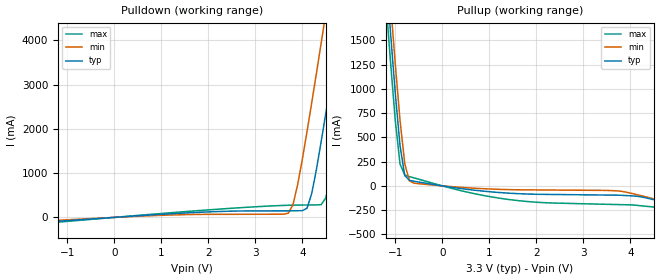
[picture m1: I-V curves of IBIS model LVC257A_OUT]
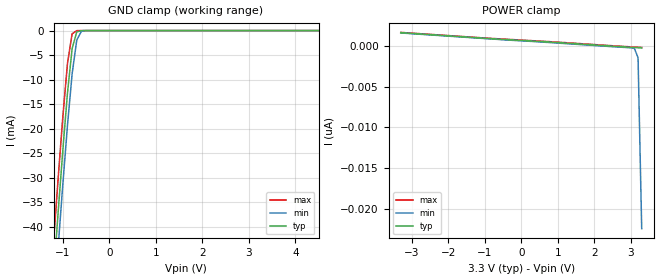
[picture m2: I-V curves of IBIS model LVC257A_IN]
|   TEXAS INSTRUMENTS INCORPORATED
|   Advanced Bus Interface Group
|   IBIS Model of LVC257A
|   Quadruple_2-Line_to_1-Line_Data_Selector/Multiplexer
|   SSOP 16-pin (DB) Package
[IBIS Ver]   2.1
[File Name]   257a.ibs
[File Rev]   1.0
[Date]   11/26/97
[Source]   File originated at Texas Instruments, Inc.
[Notes]   The following is an IBIS list for the LVC257A.
|   - All test data contained in this file are derived from
|   hspice(tm) simulations.
|   - File created by Ramzi Ammar, SLL Applications.
[Disclaimer] Property of Texas Instruments Incorporated.  Unauthorized
   reproduction and/or distribution is strictly prohibited.
   This product is protected under copyright law.
   Created 1997, (C) Copyright 1997, Texas Instruments Inc.,
   All Rights Reserved
   UNLESS THERE IS A SIGNED, WRITTEN AGREEMENT TO THE
   CONTRARY, TEXAS INSTRUMENTS ("TI") IS PROVIDING THE IBIS
   MODELS "AS IS" AND WITHOUT ANY WARRANTY, EXPRESSED OR
   IMPLIED.  TI assumes no liability for:
   1) the accuracy of the IBIS models provided to your
   company;
   2) the proper functioning of these IBIS models in your
   design or for any resulting applications; or
   3) infringement of patents, copyrights or intellectual
   property rights resulting from your use of these IBIS
   models.
   TI provides IBIS Models as a service to our customers.
   You and your company shall not distribute, sell or give
   these models to anyone else without prior written
   permission from TI.
   TI reserves the right to make changes to our products or
   to discontinue any semiconductor product or service
   without notice, and advises our customers to obtain the
   latest version of relevant information to verify, before
   placing orders, that the information being relied on is
   current.
   Please be aware that your receipt and use of the IBIS
   information provided shall serve as acceptance of these
   terms and conditions.  If you do not accept these terms,
   you should return or destroy the IBIS models and any
   other accompanying information immediately.
[Component]   LVC257A
|   (Quadruple_2-Line_to_1-Line_Data_Selector/Multiplexer)
[Manufacturer]  Texas Instruments, Inc.
[Package]
|   typ   min   max
R_pkg   0.033   0.028   0.035
L_pkg   3.97nH   3.65nH   4.58nH
C_pkg   0.34pF   0.31pF   0.37pF
[Pin]   signal_name   model_name   R_pin   L_pin   C_pin
1   A_NOT/B   LVC257A_IN   0.028   4.579nH   0.367pF
2   1A   LVC257A_IN   0.035   4.195nH   0.373pF
3   1B   LVC257A_IN   0.035   3.705nH   0.324pF
4   1Y   LVC257A_OUT   0.032   3.648nH   0.310pF
5   2A   LVC257A_IN   0.032   3.648nH   0.310pF
6   2B   LVC257A_IN   0.035   3.705nH   0.324pF
7   2Y   LVC257A_OUT   0.035   4.195nH   0.373pF
8   GND   GND   0.028   4.579nH   0.367pF
9   3Y   LVC257A_OUT   0.028   4.579nH   0.367pF
10   3B   LVC257A_IN   0.035   4.195nH   0.373pF
11   3A   LVC257A_IN   0.035   3.705nH   0.324pF
12   4Y   LVC257A_OUT   0.032   3.648nH   0.310pF
13   4B   LVC257A_IN   0.032   3.648nH   0.310pF
14   4A   LVC257A_IN   0.035   3.705nH   0.324pF
15   OE_NOT   LVC257A_IN   0.035   4.195nH   0.373pF
16   VCC   POWER   0.028   4.579nH   0.367pF
| Models and submodels in the file (2): LVC257A_OUT (Output), LVC257A_IN (Input)
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|   Model LVC257A_OUT
[Model]   LVC257A_OUT
Model_type   Output
Polarity   Inverting
|variable   typ   min   max
C_comp   5pF   NA   NA
[Voltage range]   3.3   3.0   3.6
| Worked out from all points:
|   slope of the pulldown table from 0 to 0.495 V, typ, clamps not added: 14 ohm
|   slope of the pullup table from 0 to 0.495 V, typ, clamps not added: 14.6 ohm
[Pullup]   | Note: Vtable = Vcc - Voutput
|   Voltage   I(typ)   I(min)   I(max)
-3.3V     16.91A     17.19A     16.64A
-1.2V     2.207A     2.519A     1.903A
-1.1V     1.559A     1.869A     1.259A
-1V       945.7mA    1.245A     664.8mA
-900mV    412.4mA    673.4mA    224.1mA
-800mV    106.4mA    228.5mA    111.8mA
-700mV    56.81mA    49.85mA    95.57mA
-600mV    47.48mA    27.69mA    82.06mA
1.4V      -74.65mA   -38.4mA    -139.4mA
3.8V      -96.78mA   -55.41mA   -193.4mA
4.7V      -166.8mA   -158.7mA   -231.5mA
6.6V      -409.3mA   -400.4mA   -477.6mA
[Pulldown]
|   Voltage   I(typ)   I(min)   I(max)
-3.3V     -302.9mA   -307.1mA   -301.8mA
-1.2V     -88.83mA   -65.71mA   -108.2mA
3.7V      148.2mA    92.73mA    273.4mA
3.8V      148.6mA    281.9mA    276.3mA
3.9V      149mA      735.6mA    278.3mA
4.1V      206.1mA    1.937A     279.8mA
4.2V      538.9mA    2.588A     280.4mA
4.4V      1.702A     3.929A     287.2mA
4.5V      2.352A     4.611A     438.2mA
4.8V      4.382A     6.685A     2.176A
5.1V      6.463A     8.781A     4.214A
6.6V      17.07A     19.4A      14.8A
[Ramp]
| variable   typ   min   max
dV/dt_r   1.5182E+00/3.1012E-10  1.0921E+00/4.4177E-10  1.8637E+00/2.2885E-10
dV/dt_f   1.5740E+00/2.6661E-10  1.3168E+00/3.2470E-10  1.7802E+00/2.0785E-10
|   Model LVC257A_IN
[Model]   LVC257A_IN
Model_type   Input
Polarity   Inverting
Vinl = 0.8V
Vinh = 2.0V
|variable   typ   min   max
C_comp   5pF   NA   NA
[Voltage Range]   3.3   3.0   3.6
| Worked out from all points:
|   GND clamp passes 1 mA (typ) near -0.72 V on its own axis
[POWER_Clamp]   | Note: Vtable = Vcc - Voutput
|   Voltage   I(typ)   I(min)   I(max)
-3.3V     1.569nA    1.537nA    1.605nA
3.1V      -240.8pA   -356.4pA   -183.8pA
3.2V      -265.7pA   -1.482nA   -208.7pA
3.3V      -290.6pA   -22.35nA   -233.6pA
[GND_Clamp]
|   Voltage   I(typ)   I(min)   I(max)
-3.3V     -344mA     -350.3mA   -337.8mA
-1.2V     -50.11mA   -57.21mA   -43.18mA
-1.1V     -37.01mA   -44.1mA    -30.09mA
-1V       -24.39mA   -31.38mA   -17.63mA
-900mV    -12.76mA   -19.36mA   -6.706mA
-800mV    -3.662mA   -8.823mA   -654.3uA
-700mV    -273.1uA   -1.914mA   -14.08uA
-600mV    -9.735uA   -145.1uA   -254.7nA
-500mV    -327.2nA   -7.88uA    -5.006nA
6.6V      1.569nA    1.626nA    1.515nA
